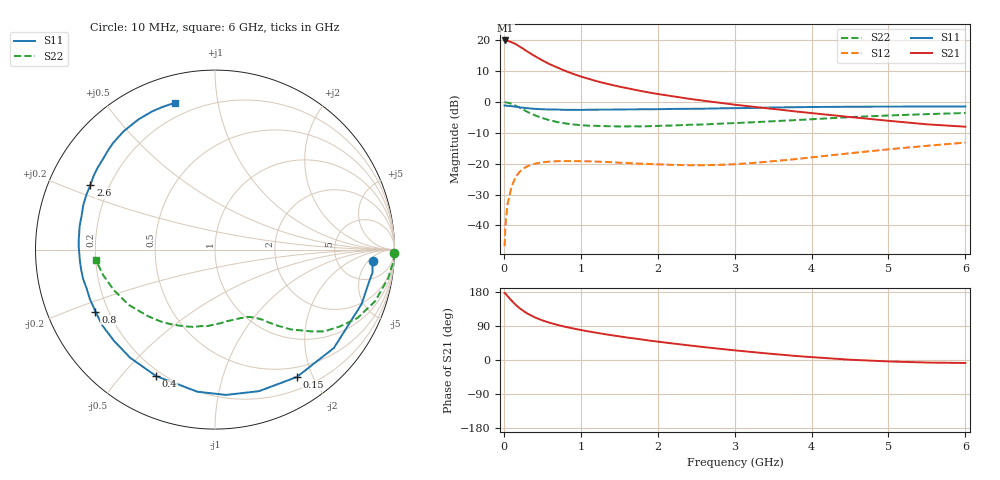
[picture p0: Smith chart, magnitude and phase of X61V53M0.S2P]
! SIEMENS Small Signal Semiconductors
! BFP193W
! Si NPN RF Bipolar Junction Transistor in SOT343
! VCE = 1.5 V  IC = 3 mA
! Common Emitter S-Parameters:  April 1994
# GHz  S  MA  R  50
!  f  S11  S21  S12  S22
! GHz  MAG  ANG  MAG  ANG  MAG  ANG  MAG  ANG
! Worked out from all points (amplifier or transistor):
!   40 points, 10 MHz to 6 GHz, reference 50 ohm
!   highest |S21| = 20.0 dB at 20 MHz (marker M1)
!   |S21| within 3 dB of that: start of sweep to 269.8 MHz
!   unconditionally stable (mu >= 1): 1.89 GHz to end of sweep
!   at 200 MHz: K = 0.11, MSG = 20.4 dB, |S12| = -22.7 dB
!   at 1.5 GHz: K = 0.79, MSG = 12.3 dB, |S12| = -19.7 dB
!   at 6 GHz: K = 1.01, MAG = 2.1 dB, |S12| = -13.1 dB
!   S11 on the Smith chart (normalised r, x): 10 MHz: 12, -7; 150 MHz: 0.36, -1.77; 400 MHz: 0.18, -0.62; 800 MHz: 0.15, -0.24; 2.6 GHz: 0.13, +0.24; 6 GHz: 0.13, +0.75
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0.01  0.8802 -4.1  9.911 176.8  0.0046 88.5  0.9996 -1.1
0.02  0.8867 -8.3  10.01 175.3  0.0094 84.0  0.9973 -4.0
0.05  0.8713 -20.4  9.858 168.1  0.0226 78.6  0.9777 -9.4
0.1  0.8597 -39.6  9.373 156.9  0.0425 68.6  0.9378 -17.8
0.15  0.8435 -57.3  8.794 146.3  0.0597 59.6  0.881 -25.6
0.2  0.826 -72.7  8.053 137.5  0.0729 52.1  0.8173 -31.6
0.25  0.812 -85.7  7.359 130.1  0.0831 45.5  0.7593 -36.9
0.3  0.7977 -97.1  6.688 123.3  0.0904 40.5  0.7013 -40.5
0.4  0.7775 -114.9  5.602 112.8  0.0998 32.0  0.6128 -46.5
0.5  0.7659 -128.1  4.761 104.5  0.1056 26.5  0.5512 -50.4
0.6  0.7584 -138.0  4.101 98.0  0.1085 22.0  0.5059 -53.5
0.7  0.7568 -146.3  3.623 92.5  0.1099 19.0  0.4736 -55.7
0.8  0.75 -152.6  3.2 87.5  0.1106 16.5  0.4511 -58.2
1.1  0.7527 -167.3  2.393 75.5  0.1095 11.7  0.4148 -64.6
1.3  0.7554 -175.0  2.04 68.6  0.1073 10.2  0.4078 -69.2
1.6  0.7615 175.9  1.687 59.3  0.103 10.0  0.4039 -75.9
2.2  0.7751 161.1  1.241 43.5  0.0959 14.3  0.4174 -90.6
2.6  0.7822 152.5  1.052 34.1  0.0946 20.2  0.434 -100.7
3.2  0.8025 141.0  0.852 21.6  0.1021 30.2  0.4685 -115.3
4.5  0.8415 120.4  0.573 0.8  0.1481 40.2  0.5704 -147.2
5.5  0.8469 110.2  0.436 -6.7  0.1955 38.1  0.6385 -167.0
6  0.8478 105.4  0.399 -7.9  0.2204 35.8  0.6658 -174.8
